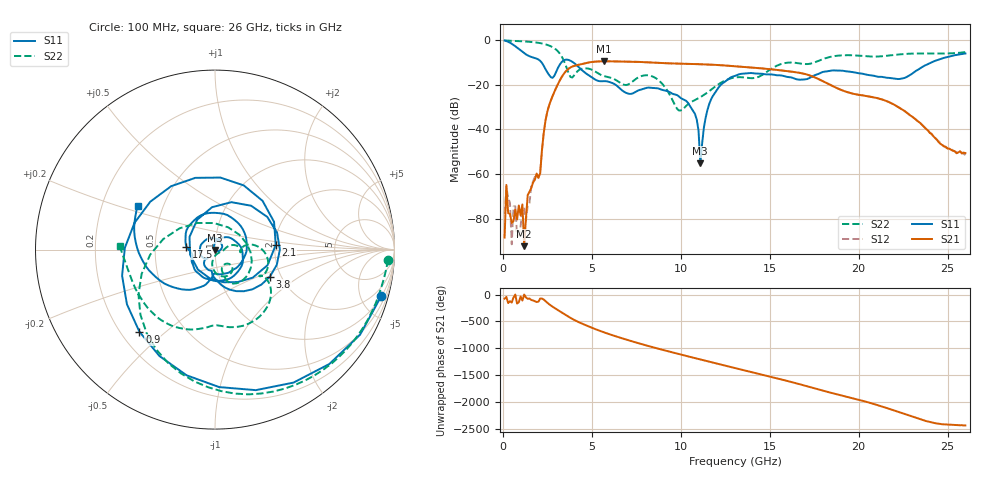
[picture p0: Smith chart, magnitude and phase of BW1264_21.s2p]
!Keysight Technologies,N5245B,MY57181159,A.13.60.06
!Date: Friday, December 18, 2020 23:53:01
!Correction: S11(Full 2 Port(1,2))
!S21(Full 2 Port(1,2))
!S12(Full 2 Port(1,2))
!S22(Full 2 Port(1,2))
!S2P File: Measurements: S11, S21, S12, S22:
# Hz S  dB  R 50
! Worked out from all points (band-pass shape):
!   260 points, 100 MHz to 26 GHz, reference 50 ohm
!   highest |S21| = -9.61 dB at 5.7 GHz (marker M1); lowest = -92.0 dB at 1.2 GHz (marker M2)
!   |S21| within 3 dB of the highest: 3.753 GHz to 14.33 GHz (10.57 GHz wide, 117 % of centre)
!   lowest |S11| = -55.0 dB at 11.1 GHz (marker M3), VSWR 1.00, Z = 50.1 - j0.139 ohm
!   |S11| at or under -10 dB: 2.167 GHz to 3.299 GHz (1.132 GHz wide, 41.4 % of centre); 3.938 GHz to 24.12 GHz (20.18 GHz wide, 144 % of centre)
!   |S22| runs from -31.6 to -0.3 dB; largest |S21 - S12| = 0.0005
!   S11 on the Smith chart (normalised r, x): 100 MHz: 1.04, -7.19; 900 MHz: 0.28, -0.41; 2.1 GHz: 2.02, +0.12; 3.8 GHz: 1.76, -0.60; 17.5 GHz: 0.72, +0.03; 26 GHz: 0.36, +0.23
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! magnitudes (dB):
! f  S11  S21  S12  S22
! 100 MHz  -0.3  -88.2  -77.7  -0.3
! 200 MHz  -0.6  -64.7  -65.4  -0.4
! 300 MHz  -0.9  -77.3  -70.6  -0.4
! 500 MHz  -1.8  -81.6  -91.2  -0.5
! 900 MHz  -4.1  -73.9  -87.3  -0.6
! 1.2 GHz  -6.0  -92.0  -74.9  -0.7
! 2.1 GHz  -9.4  -59.5  -58.4  -1.5
! 2.6 GHz  -15.7  -29.3  -29.3  -2.6
! 3.8 GHz  -9.3  -12.4  -12.4  -16.6
! 4.5 GHz  -13.9  -10.7  -10.8  -12.8
! 5.7 GHz  -18.5  -9.6  -9.6  -16.2
! 8.8 GHz  -21.9  -10.3  -10.3  -18.4
! 9.9 GHz  -25.3  -10.6  -10.7  -31.6
! 10.8 GHz  -33.1  -10.8  -10.8  -26.8
! 11 GHz  -40.5  -10.9  -10.9  -26.0
! 11.1 GHz  -55.0  -10.9  -10.9  -25.6
! 11.7 GHz  -26.6  -11.1  -11.1  -22.3
! 13.1 GHz  -16.0  -11.8  -11.8  -16.7
! 17.4 GHz  -16.3  -16.3  -16.3  -10.4
! 17.5 GHz  -15.9  -16.7  -16.6  -10.2
! 21.7 GHz  -17.0  -27.8  -27.8  -7.0
! 26 GHz  -6.1  -50.5  -51.4  -5.5
